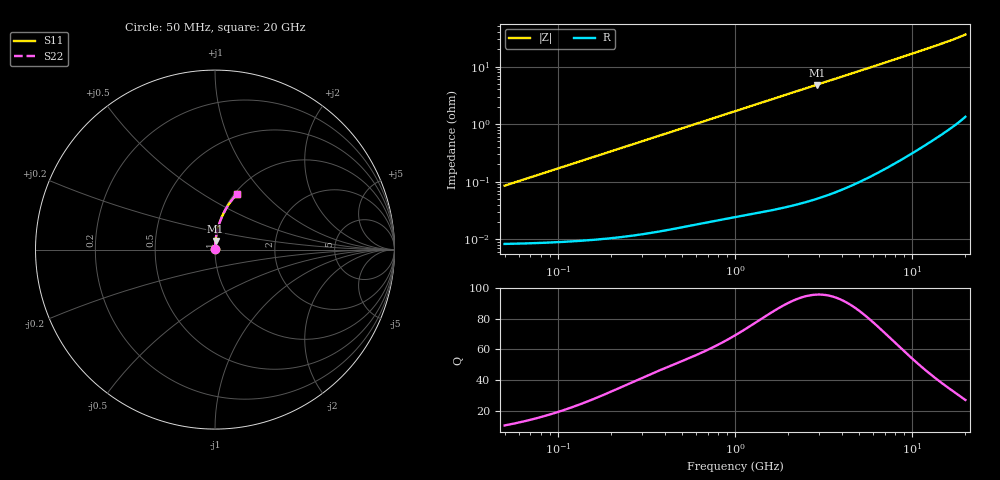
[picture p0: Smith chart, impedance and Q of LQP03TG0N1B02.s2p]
!Murata Part Number: LQP03TG0N1B02
!These Parameters are Measured in Series Mode Connection
!  o--[Z]--o
!Port1  Port2
!  o-------o
!Freq. Start=50[MHz] Stop=20[GHz], 401[Steps]
# Hz S RI R 50
!Freq.(Hz) S11(Real) S11(Imag) S21(Real) S21(Imag) S12(Real) S12(Imag) S22(Real) S22(Imag)
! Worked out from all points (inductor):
!   401 points, 50 MHz to 20 GHz, reference 50 ohm
!   read as one part in series: L = 269 pH near 51.52 MHz
!   highest Q = 95.9 at 2.896 GHz (marker M1), where L = 265 pH
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5e7  8.34e-05 0.000847  0.9999 -0.000847  0.9999 -0.000847  8.34e-05 0.000847
5.152053e7  8.36e-05 0.000872  0.9999 -0.000872  0.9999 -0.000872  8.36e-05 0.000872
1.364002e8  9.93e-05 0.0023  0.9999 -0.0023  0.9999 -0.0023  9.93e-05 0.0023
3.721004e8  0.000175 0.00625  0.9998 -0.00625  0.9998 -0.00625  0.000175 0.00625
6.380365e8  0.0003 0.0107  0.9997 -0.0107  0.9997 -0.0107  0.0003 0.0107
1e9  0.000519 0.0167  0.9995 -0.0167  0.9995 -0.0167  0.000519 0.0167
1.714689e9  0.00114 0.0285  0.9989 -0.0285  0.9989 -0.0285  0.00114 0.0285
2.728004e9  0.00252 0.0452  0.9975 -0.0452  0.9975 -0.0452  0.00252 0.0452
2.896447e9  0.00281 0.048  0.9972 -0.048  0.9972 -0.048  0.00281 0.048
3.792786e9  0.00462 0.0627  0.9954 -0.0627  0.9954 -0.0627  0.00462 0.0627
4.81993e9  0.00729 0.0795  0.9927 -0.0795  0.9927 -0.0795  0.00729 0.0795
6.034176e9  0.0112 0.0992  0.9888 -0.0992  0.9888 -0.0992  0.0112 0.0992
7.442007e9  0.0169 0.1218  0.9831 -0.1218  0.9831 -0.1218  0.0169 0.1218
8.644534e9  0.0227 0.1409  0.9773 -0.1409  0.9773 -0.1409  0.0227 0.1409
1.004137e10  0.0304 0.1627  0.9696 -0.1627  0.9696 -0.1627  0.0304 0.1627
1.166392e10  0.0408 0.1876  0.9592 -0.1876  0.9592 -0.1876  0.0408 0.1876
1.334722e10  0.0533 0.2129  0.9467 -0.2129  0.9467 -0.2129  0.0533 0.2129
1.482269e10  0.0656 0.2347  0.9344 -0.2347  0.9344 -0.2347  0.0656 0.2347
1.646126e10  0.0812 0.2587  0.9188 -0.2587  0.9188 -0.2587  0.0812 0.2587
1.800918e10  0.098 0.2815  0.902 -0.2815  0.902 -0.2815  0.098 0.2815
1.940974e10  0.116 0.3028  0.884 -0.3028  0.884 -0.3028  0.116 0.3028
2e10  0.1247 0.3123  0.8753 -0.3123  0.8753 -0.3123  0.1247 0.3123
